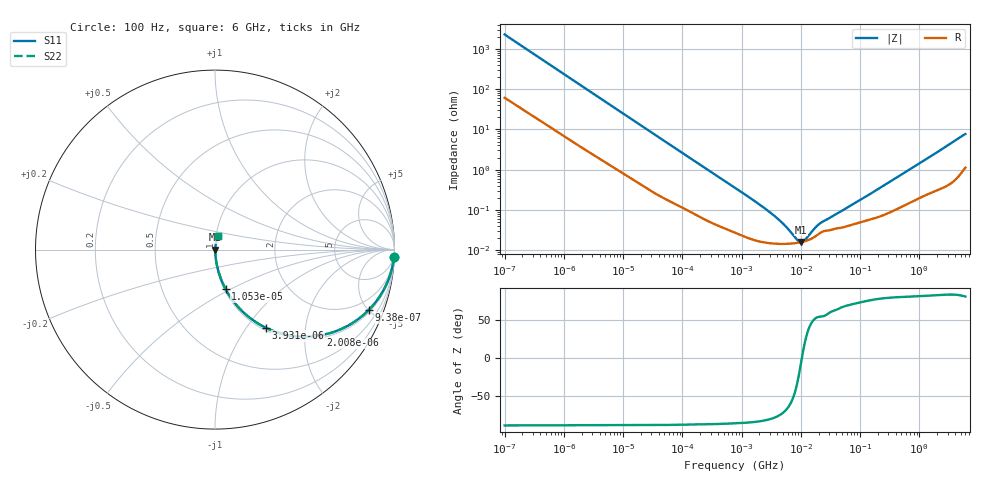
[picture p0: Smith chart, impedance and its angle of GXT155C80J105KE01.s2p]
!Murata Part Number: GXT155C80J105KE01
!These Parameters are Measured in Series Mode Connection
!Data Generated on Jan 08, 2026
!  o--ll--o
!Port1  Port2
!  o------o
!Operation Temp=25[degC], DC Bias Voltage=0[V]
!Freq. Start=100[Hz] Stop=6[GHz] 401[Steps]
# Hz S RI R 50
!Freq.(Hz) S11(Real) S11(Imag) S21(Real) S21(Imag) S12(Real) S12(Imag) S22(Real) S22(Imag)
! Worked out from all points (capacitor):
!   401 points, 100 Hz to 6 GHz, reference 50 ohm
!   read as one part in series: C = 695 nF near 109 Hz
!   lowest |Z| = 16 mohm at 9.942 MHz (marker M1)
!   series resonance near 10.4 MHz, so ESL is about 340 pH
!   S11 on the Smith chart (normalised r, x): 100 Hz: 2, -46; 938 Hz: 1.15, -5.06; 2.008 kHz: 1.07, -2.39; 3.931 kHz: 1.04, -1.24; 10.53 kHz: 1.02, -0.47; 6 GHz: 1.02, +0.15
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100  0.9969 -0.0437  0.00309 0.0437  0.00309 0.0437  0.9969 -0.0437
335  0.976 -0.1398  0.024 0.1398  0.024 0.1398  0.976 -0.1398
600  0.9332 -0.2359  0.0668 0.2359  0.0668 0.2359  0.9332 -0.2359
938  0.8577 -0.3352  0.1423 0.3352  0.1423 0.3352  0.8577 -0.3352
1342  0.7536 -0.4166  0.2464 0.4166  0.2464 0.4166  0.7536 -0.4166
2008  0.5867 -0.4779  0.4133 0.4779  0.4133 0.4779  0.5867 -0.4779
2748  0.4386 -0.4814  0.5614 0.4814  0.5614 0.4814  0.4386 -0.4814
3931  0.2834 -0.4355  0.7166 0.4355  0.7166 0.4355  0.2834 -0.4355
6151  0.1454 -0.3371  0.8546 0.3371  0.8546 0.3371  0.1454 -0.3371
10527  0.0591 -0.2202  0.9409 0.2202  0.9409 0.2202  0.0591 -0.2202
19704  0.0201 -0.1245  0.9799 0.1245  0.9799 0.1245  0.0201 -0.1245
40335  0.00623 -0.0627  0.9938 0.0627  0.9938 0.0627  0.00623 -0.0627
774597  0.000284 -0.00354  0.9997 0.00354  0.9997 0.00354  0.000284 -0.00354
3549919  0.000147 -0.000706  0.9999 0.000706  0.9999 0.000706  0.000147 -0.000706
5311619  0.000144 -0.000395  0.9999 0.000395  0.9999 0.000395  0.000144 -0.000395
8692127  0.000152 -9.81e-05  0.9998 9.81e-05  0.9998 9.81e-05  0.000152 -9.81e-05
9941735  0.000158 -2.43e-05  0.9998 2.43e-05  0.9998 2.43e-05  0.000158 -2.43e-05
1.189169e7  0.000169 7.32e-05  0.9998 -7.32e-05  0.9998 -7.32e-05  0.000169 7.32e-05
1.555665e7  0.000198 0.000222  0.9998 -0.000222  0.9998 -0.000222  0.000198 0.000222
2.225763e7  0.000281 0.000403  0.9997 -0.000403  0.9997 -0.000403  0.000281 0.000403
3.124326e8  0.000879 0.00486  0.9991 -0.00486  0.9991 -0.00486  0.000879 0.00486
6e9  0.0167 0.074  0.9833 -0.074  0.9833 -0.074  0.0167 0.074
